FUNCTION_BLOCK FB71
TITLE =Get Position Profile
//*****************************************************************************
//* maxon motor ag
//* R&D
//* all rights reserved
//*****************************************************************************
//* Summary:  gets the position profile
//*
//* Remarks:
//*
//* Created under: STEP7 REV5.2+SP1
//*****************************************************************************
//* History:
//* 19.05.2004 | INA   first release
//*
//*
//*****************************************************************************
//

AUTHOR:INA
FAMILY:ProPosMo
NAME:GetPosPr
VERSION:00.01


VAR_INPUT

Read : BOOL //A rising edge start the command

  NodeID : BYTE //Adress of the maxon device

END_VAR
VAR_OUTPUT
  Done : BOOL //Data valid flag is TRUE if data were available

  Err : BOOL //Error flag is TRUE if an Error has occured, see ErrNo for more details

  ErrNo : DINT //Contains detailed error information

  ProfileVelocity : DWORD //Position Profile Velocity

  ProfileAcceleration : DWORD //Position Profile Acceleration

  ProfileDeceleration : DWORD //Position Profile Deceleration

END_VAR
VAR
  xEdgeMerker : BOOL //Edge Merker

  xEdgeFlag : BOOL //Edge Flag

  xStep : INT
END_VAR

BEGIN

NETWORK
TITLE = Activate the service function
//

// SDO Read "Get Position Profile"

       U    #Read
       FP   #xEdgeFlag                   // recognize a positiv edge of the Read signal
       =    #xEdgeMerker                 // and set the xEdgeMerker for one cycle to true

       L    #xStep
       L    0
       ==I
       U    #xEdgeMerker
       SPB  nstp                         // iStep = 1 -> fnc1

       L    #xStep                       // jump list
       SPL  List
       SPA  rdef
       SPA  fnc1
       SPA  fncE
List  :SPA  rdef

rdef  :NOP  0
       R    #Done                        // reset Done
       R    #Err                         // reset Error
       L    0
       T    #xStep                       // iStep = 0
       SPA  end

fnc1  :NOP  0
       CALL FC1
         NodeID:=#NodeID
         Index:=DW#16#00006081
         SubIndex:=DW#16#00000000
         RET_VAL:=#Done
         Err:=#Err
         ErrNo:=#ErrNo

       L    DB219.DBD10
       T    #ProfileVelocity

       L    1
       U    #Err
       SPB  fncE

       NOP  0
       CALL FC1
         NodeID:=#NodeID
         Index:=DW#16#00006083
         SubIndex:=DW#16#00000000
         RET_VAL:=#Done
         Err:=#Err
         ErrNo:=#ErrNo

       L    DB219.DBD10
       T    #ProfileAcceleration

       L    1
       U    #Err
       SPB  fncE

       NOP  0
       CALL FC1
         NodeID:=#NodeID
         Index:=DW#16#00006084
         SubIndex:=DW#16#00000000
         RET_VAL:=#Done
         Err:=#Err
         ErrNo:=#ErrNo

       L    DB219.DBD10
       T    #ProfileDeceleration

fncE  :NOP  0
       L    0
       T    #xStep
       SPA  end

nstp  :NOP  0
       L    #xStep
       INC            1
       T    #xStep

end   :NOP  0
END_FUNCTION_BLOCK
